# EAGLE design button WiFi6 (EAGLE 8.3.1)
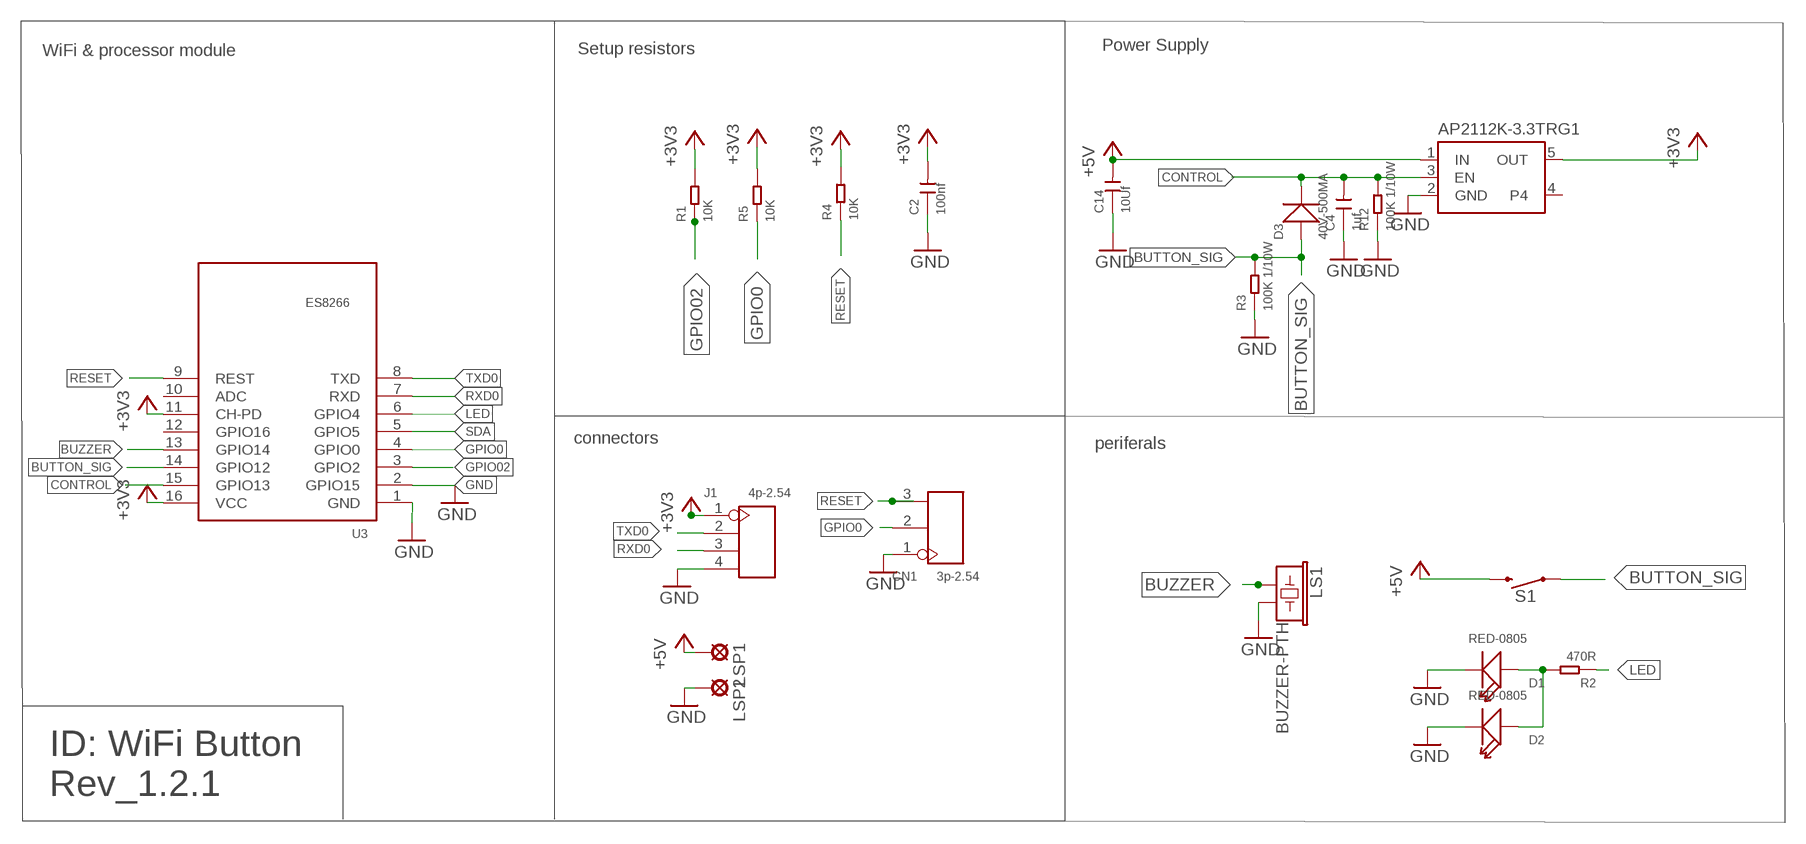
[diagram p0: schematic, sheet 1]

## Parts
AP2112K-3.3TRG1  SPX3819  VREG_SOT23-5  [SOT23-5]
C2  100nf  CERAMIC-100NF-50V-10%-X7R(0603)  [C0603]
C4  1uf  CERAMIC-1UF-25V-10%-X7R(0603)  [C0603]
C14  10Uf  CERAMIC-100NF-50V-10%-X7R(0603)  [C0603]
CN1  3p-2.54  DIP-BLACK-MALE-HEADER-VERT(3P-2.54)  [H3-2.54]
D1  RED-0805  SMD-LED-CLEAR-RED(0805)  [LED-0805]
D2  RED-0805  SMD-LED-CLEAR-RED(0805)  [LED-0805]
D3  40V-500MA  SMD-DIODE-SCHOTTKY-40V-500MA(SOD-123)  [SOD-123]
J1  4p-2.54  DIP-BLACK-FEMALE-HEADER-VERT(4P-2.54)  [H4-2.54]
LS1  BUZZER-PTH  [BUZZER-12MM]
LSP1  SE11  [SE11]
LSP2  SE11  [SE11]
R1  10K  SMD-RES-10K-1%-1/10W(0603)  [R0603]
R2  470R  SMD-RES-470R-5%-1/10W(0603)  [R0603]
R3  100K 1/10W  SMD-RES-100K-5%-1/10W(0603)  [R0603]
R4  10K  SMD-RES-10K-1%-1/10W(0603)  [R0603]
R5  10K  SMD-RES-10K-1%-1/10W(0603)  [R0603]
R12  100K 1/10W  SMD-RES-100K-5%-1/10W(0603)  [R0603]
S1  MOMENTARY-SWITCH-SPST-SMD-6.2MM-TALL  [TACTILE_SWITCH_SMD_6.2MM_TALL]
U3  ES8266  MOUDLE-WIFI-ESP8266-AKX(16P-24X16MM)  [LGA16-2.0-24X16MM]

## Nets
+3V3: AP2112K-3.3TRG1.5(OUT) C2.2 J1.1 R1.2 R4.2 R5.2 U3.11(CH-PD) U3.16(VCC)
+5V: AP2112K-3.3TRG1.1(IN) C14.2 LSP1.MP S1.B2
BUTTON_SIG: D3.+ R3.2 S1.A2 U3.14(GPIO12)
BUZZER: LS1.+ U3.13(GPIO14)
CONTROL: AP2112K-3.3TRG1.3(EN) C4.2 D3.- R12.2 U3.15(GPIO13)
GND: AP2112K-3.3TRG1.2(GND) C2.1 C4.1 C14.1 CN1.1 D1.- D2.- J1.4 LS1.- LSP2.MP R3.1 R12.1 U3.1(GND) U3.2(GPIO15)
GPIO0: CN1.2 R5.1 U3.4(GPIO0)
GPIO02: R1.1 U3.3(GPIO2)
LED: R2.1 U3.6(GPIO4)
N$2: D1.+ D2.+ R2.2
RESET: CN1.3 R4.1 U3.9(REST)
RXD0: J1.3 U3.7(RXD)
SDA: U3.5(GPIO5)
TXD0: J1.2 U3.8(TXD)
Unconnected: AP2112K-3.3TRG1.4 U3.10(ADC) U3.12(GPIO16)

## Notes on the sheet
- Setup resistors | Power Supply
- WiFi & processor module
- connectors
- periferals
- ID: WiFi Button 
  Rev_1.2.1

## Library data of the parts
AP2112K-3.3TRG1 = microbuilder:VREG_SOT23-5: SOT23-5 Fixed Voltage Regulators Part Current Out V Out V In V Dropout θJA (°C/W) TJ (°C) Digikey Part No. ADP121 150mA 3.3V 3.4-5.5V 0.09V @ 150mA -- -- ADP121-AUJZ33R7CT-ND ADP121 150mA 3.0V 3.1-5.5V 0.09V @ 150mA -- -- ADP121-AUJZ30R7CT-ND ADP122 300mA 3.3V 3.4-5.5V 0.085V @ 300mA -- --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
C2 = Seeed-Capacitor:CERAMIC-100NF-50V-10%-X7R(0603): 302010138; MPN: CC0603KRX7R9BB104
C4 = Seeed-Capacitor-2016:CERAMIC-1UF-25V-10%-X7R(0603): 302010139; MPN: CC0603KRX7R8BB105
C14 = Seeed-OPL-Capacitor:CERAMIC-100NF-50V-10%-X7R(0603): 302010138; MPN: CC0603KRX7R9BB104; VALUE: 100nf
CN1 = Seeed-Connector -2016:DIP-BLACK-MALE-HEADER-VERT(3P-2.54): 320020079
D1 D2 = Seeed-LED-2016:SMD-LED-CLEAR-RED(0805): 304090046; MPN: 17-215SURC/S530-A2/TR8
D3 = Seeed-Diode:SMD-DIODE-SCHOTTKY-40V-500MA(SOD-123): 304020012; MPN: B0540W
J1 = Seeed-Connector:DIP-BLACK-FEMALE-HEADER-VERT(4P-2.54): 320030017; MPN: F185-1104A1BSYA1
LS1 = SparkFun-Electromechanical:BUZZER: Buzzer; PROD_ID: COMP-08253; SF_SKU: COM-07950
LSP1 LSP2 = solpad:SE11: SOLDER PAD
R1 R4 R5 = Seeed-Resistor-2016:SMD-RES-10K-1%-1/10W(0603): 301010299; MPN: RC0603FR-0710KL
R2 = Seeed-Resistor-2016:SMD-RES-470R-5%-1/10W(0603): 301010088; MPN: RC0603JR-07470RL
R3 R12 = Seeed-Resistor-2016:SMD-RES-100K-5%-1/10W(0603): 301010089; MPN: RC0603JR-07100KL
S1 = SparkFun-Switches:MOMENTARY-SWITCH-SPST: Momentary Switch (Pushbutton) - SPST; PROD_ID: SWCH-11966; SF_SKU: COM-12992
U3 = Seeed-OPL-Moudle:MOUDLE-WIFI-ESP8266-AKX(16P-24X16MM): 317060011; MPN: ES8266

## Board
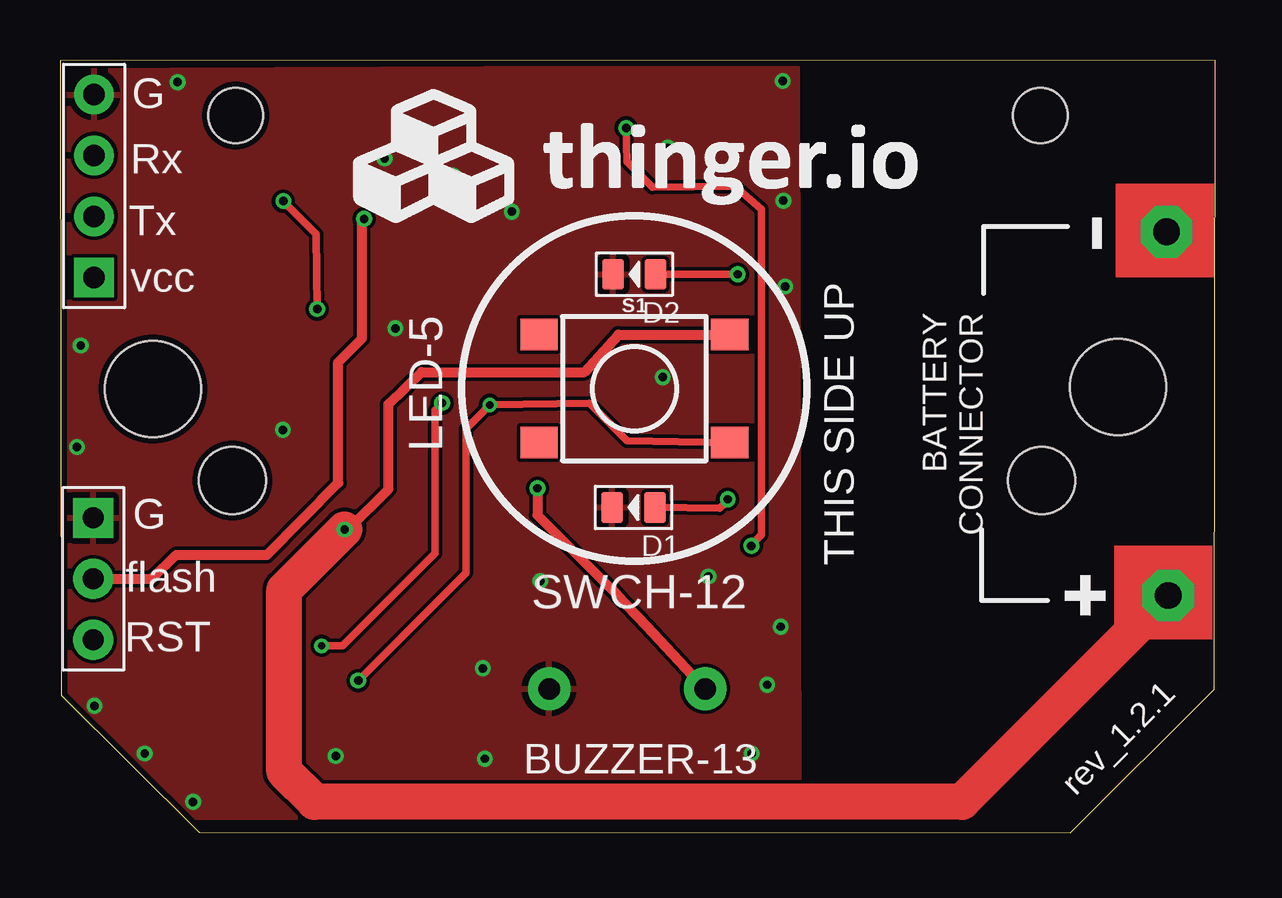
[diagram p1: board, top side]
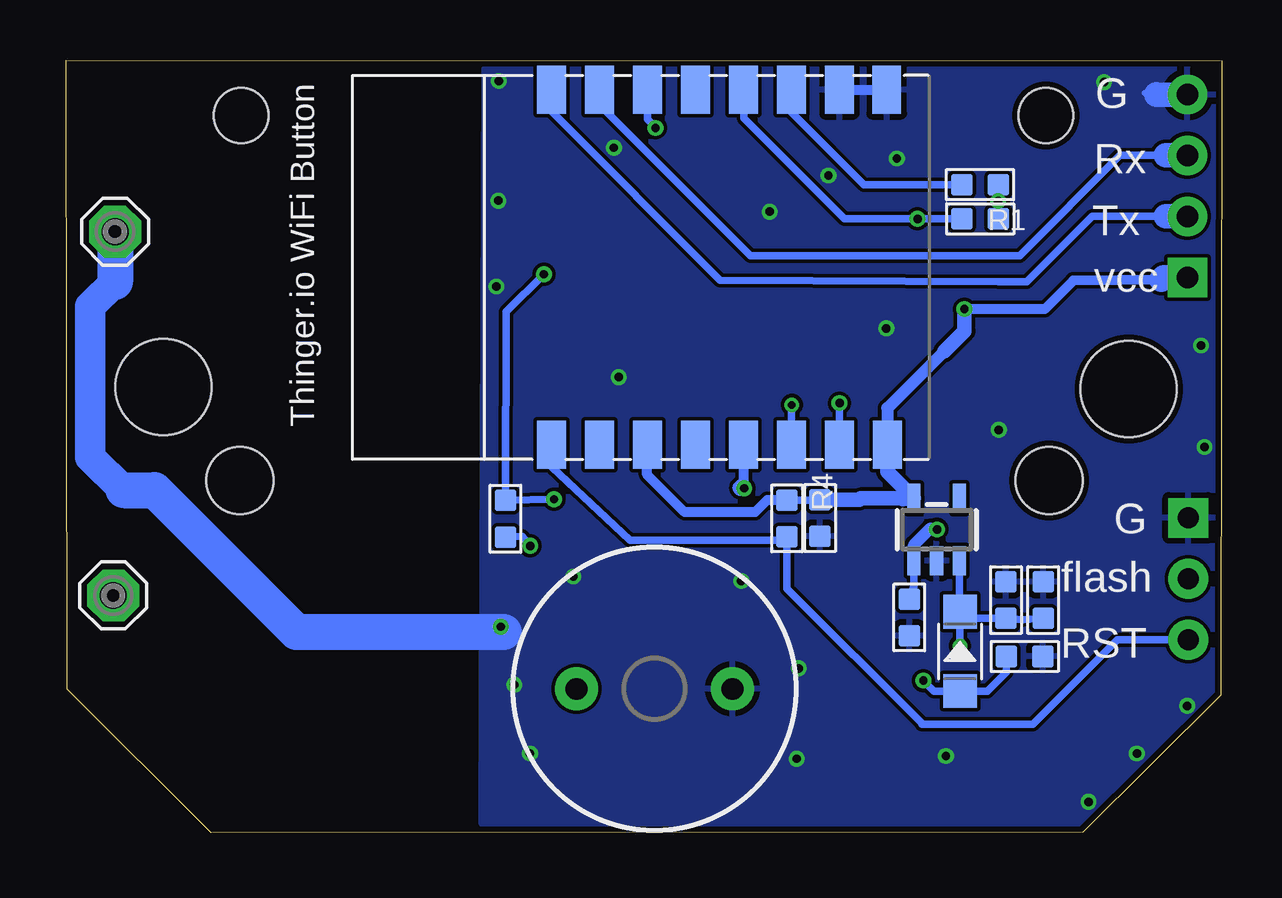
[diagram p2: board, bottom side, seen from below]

Size 48.15 x 32.2 mm. Coordinates in mm from the lower left corner, seen from the top.
Outline: 0,32.18 0.04,5.74 5.79,0.02 42.11,0 48.11,5.99 48.15,32.2 0,32.18
Copper layers (1*16): Top 0.035mm / dielectric 1.5mm / Bottom 0.035mm
Design rules "SeeedStudio_2layer_DRU_no_angle_20140221": minimum track width 6mil, minimum drill 12mil, track to track 6mil, track to pad 6mil, pad to pad 6mil, via to via 6mil, smd to smd 0mil, copper to edge 10mil, drill to drill 10mil, minimum pad ring 10mil, minimum via ring 6mil, stop-mask expansion 2mil, vias tented up to drill 100mil, thermal gap 10mil
Holes 2.8 mm at 7.19,14.69 40.92,14.69
Holes 2.29 mm at 7.33,29.89 40.86,29.89
Holes 4 mm at 3.87,18.5 44.11,18.57

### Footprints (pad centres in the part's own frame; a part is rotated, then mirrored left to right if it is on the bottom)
SOT23-5 = smd 0.55 x 1.2: 1 -0.95,-1.3; 2 0,-1.3; 3 0.95,-1.3; 4 0.95,1.3; 5 -0.95,1.3
C0603 = smd 0.889 x 0.889: 1 0,0.762; 2 0,-0.762
H3-2.54 = drill 0.889 pad 1.651 square: 1 0,2.54 | drill 0.889 pad 1.651: 2 0,0; 3 0,-2.54
LED-0805 = smd 0.889 x 1.27: + -0.889,0; - 0.889,0
SOD-123 = smd 1.397 x 1.397: + -1.651,0; - 1.651,0
H4-2.54 = drill 0.889 pad 1.651 square: 1 0,3.81 | drill 0.889 pad 1.651: 2 0,1.27; 3 0,-1.27; 4 0,-3.81
BUZZER-12MM = drill 0.9 pad 1.778: + 3.25,0; - -3.25,0
SE11 = drill 1.118 pad 2.159 octagon: MP 0,0
R0603 = smd 0.889 x 0.889: 1 0,0.762; 2 0,-0.762
TACTILE_SWITCH_SMD_6.2MM_TALL = smd 1.55 x 1.3: A1 -3.975,-2.25; A2 3.975,-2.25; B1 -3.975,2.25; B2 3.975,2.25
LGA16-2.0-24X16MM = smd 2 x 1.2: 1 7.4,-10.27; 2 7.4,-8.3; 3 7.4,-6.3; 4 7.4,-4.3; 5 7.4,-2.3; 6 7.4,-0.3; 7 7.4,1.7; 8 7.4,3.7; 9 -7.4,3.7; 10 -7.4,1.7; 11 -7.4,-0.3; 12 -7.4,-2.3; 13 -7.4,-4.3; 14 -7.4,-6.3; 15 -7.4,-8.3; 16 -7.4,-10.3

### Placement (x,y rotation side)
AP2112K-3.3TRG1  11.88,12.64 0 bottom
C2  16.74,13.12 180 bottom
C4  8.99,9.7 0 bottom
C14  13.01,8.98 180 bottom
CN1  1.39,10.59 0 top
D1  23.9,13.56 180 top
D2  23.94,23.28 180 top
D3  10.9,7.56 90 bottom
J1  1.42,26.96 180 top
LS1  23.64,6 180 bottom
LSP1  46.2,9.89 0 bottom
LSP2  46.12,25.05 0 bottom
R1  10.07,27.01 90 bottom
R2  29.86,13.09 180 bottom
R3  8.21,7.35 270 bottom
R4  18.11,13.1 180 bottom
R5  10.06,25.58 90 bottom
R12  7.44,9.7 0 bottom
S1  23.94,18.51 0 top
U3  24.23,23.57 90 bottom

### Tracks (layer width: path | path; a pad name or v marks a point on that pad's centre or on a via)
+3V3  (via drill 0.35)
  Top 0.305: v10.72,21.83 10.68,24.95 v9.31,26.32
  Bottom 0.203: U3.16 13.93,15.61
  Bottom 0.254: 2.95,22.95 J1.1
  Bottom 0.305: C2.2 16.76,13.86 16.76,13.87 R4.2 | U3.16 13.93,15.56 | R5.2 v9.31,26.32 R1.2
  Bottom 0.406: 2.51,23.05 6.19,23.01 7.37,21.83 v10.72,21.83 | R4.2 18.95,13.87 19.45,13.37 22.38,13.37 23.94,14.93 23.94,16.16 U3.11
  Bottom 0.508: U3.16 13.93,17.7 11.56,20.07 | v10.72,21.83 10.73,21.49
  Bottom 0.61: 14.23,15.86 U3.16 13.93,15.04 AP2112K-3.3TRG1.5 | AP2112K-3.3TRG1.5 13.28,13.89 | C2.2 15.1,13.88 15.05,13.94 AP2112K-3.3TRG1.5 | 11.56,20.07 10.72,20.91 v10.72,21.83
  Bottom 1.016: J1.1 2.41,23.15 2.51,23.05
+5V  (via drill 0.35)
  Top 0.406: v11.86,12.65 12.02,12.65 13.69,14.32 13.69,17.87 15.06,19.2 21.86,19.2 23.27,20.76 S1.B2
  Top 1.016: 45.5,9.19 LSP1.MP
  Top 1.5: LSP1.MP 37.6,1.29 10.61,1.29 9.35,2.55 9.35,10.13 v11.86,12.65
  Bottom 0.305: AP2112K-3.3TRG1.1 12.83,10.27 C14.2
  Bottom 0.508: AP2112K-3.3TRG1.1 12.82,11.35 12.82,12 12.13,12.68 v11.86,12.65
BUTTON_SIG  (via drill 0.3, 0.35)
  Top 0.305: 27.74,16.57 S1.A2 23.64,16.34 22.07,17.91 v17.92,17.84 16.93,16.85 16.93,10.85 v12.43,6.35
  Bottom 0.305: v12.43,6.35 12,5.91 D3.+ | D3.+ 11.02,5.87 | D3.+ | R3.2 8.97,6.7 9.77,5.9 10.89,5.9 D3.+ | U3.14 17.93,17.82 v17.92,17.84
BUZZER  (via drill 0.35)
  Top 0.406: 23.2,9.94 22.95,10.21 | 23.2,9.94 24.48,8.61 LS1.+ | v19.9,14.36 19.9,13.24 23.2,9.94
  Bottom 0.406: U3.13 19.93,14.29 19.94,14.28 arc323 v19.9,14.36
CONTROL  (via drill 0.3, 0.35)
  Top 0.305: v15.93,17.91 15.64,17.62 15.64,11.66 11.78,7.8 v10.91,7.79
  Bottom 0.305: U3.15 15.93,17.76 15.85,17.84 v15.93,17.91 | 7.49,8.89 R12.2 8.28,8.89 C4.2 10.62,8.94 D3.- | D3.- 10.9,8.68 v10.91,7.79 | AP2112K-3.3TRG1.3 10.93,9.24 D3.-
GND  (via drill 0.35)
  Bottom 0.254: 2.73,30.78 3.22,30.82
  Bottom 0.406: U3.2 U3.1
  Bottom 1.016: J1.4 2.72,30.77 2.73,30.78
  Bottom 1.27: 46.12,22.96 47.15,21.94 47.15,15.66 45.77,14.28
  Bottom 1.5: LSP2.MP 46.12,22.96 | 45.77,14.28 44.48,14.28 38.57,8.38 29.92,8.38
  other vias: 30.15,26.34 30.13,31.33 13.53,28.09 18.84,25.88 13.98,21.02 30.23,22.76 17.63,6.86 17.71,3.09 28.83,3.31 16.39,27.39 25.33,28.55 11.49,3.2 3.53,3.31 27.03,10.68 20.02,10.49 25.12,18.99 30.04,8.59 9.29,16.79 5.55,1.29 1.44,5.29 0.71,16.08 0.86,20.31 4.9,31.28 29.48,6.17
  pour Bottom: 0.19,32 0.32,0.36 30.84,0.36 30.73,31.84
  pour Top: 0.23,31.73 0.12,5.85 5.62,0.66 30.81,0.71 30.73,31.87
GPIO0  (via drill 0.35)
  Top 0.305: 12.51,25.47 12.69,25.64
  Top 0.406: v12.68,25.59 12.69,25.6 12.69,25.64 12.59,25.54 12.59,20.61 11.6,19.62 11.6,14.59 8.63,11.58 4.85,11.58 3.83,10.59 CN1.2
  Bottom 0.305: R5.1 12.54,25.59 v12.68,25.59 15.68,25.59 15.69,25.59 | 19.89,30.92 U3.4 19.91,30.94 19.91,29.77 15.73,25.59 15.69,25.59 | 15.69,25.59 15.54,25.59
GPIO02
  Bottom 0.305: R1.1 14.91,27.01 18,30.1 18,30.9 U3.3
LED  (via drill 0.35)
  Top 0.305: v23.6,29.37 23.64,27.96 24.7,26.9 28.13,26.93 29.24,25.98 29.24,12.42 28.82,12 v28.82,11.96
  Bottom 0.305: U3.6 23.93,29.74 v23.6,29.37 23.45,29.26 | v28.82,11.96 29.16,12.36 R2.1
N$2  (via drill 0.35)
  Top 0.305: D1.+ 27.49,13.52 27.87,13.87 v27.83,13.9 | D2.+ v28.25,23.28
  Bottom 0.305: v28.25,23.28 29.82,21.71 R2.2 v27.83,13.9
RESET
  Bottom 0.305: U3.9 27.9,16.14 27.9,15.24 24.67,12.19 18.27,12.19 R4.1 18.11,10.17 12.5,4.56 12.5,4.53 7.86,4.53 4.35,8.05 CN1.3
RXD0
  Bottom 0.254: J1.3
  Bottom 0.305: U3.7 25.96,30.94 25.87,30.85 25.8,30.21 19.63,24.05 8.42,24.05 4.24,28.23 J1.3
  Bottom 1.016: J1.3 2.34,28.23
TXD0
  Bottom 0.305: 27.91,30.62 27.91,30.04 20.91,23.04 9.31,22.96 8.11,22.96 5.39,25.69 2.08,25.69 | 27.91,30.62 27.91,30.95 U3.8 | 27.93,30.6 27.91,30.62
  Bottom 1.016: J1.2 2.08,25.69 2.33,25.69
(copper drawn outside any net)
  shapes: Top area x2

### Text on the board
tNames: G | Rx | Tx | - | vcc | LED-5 | BATTERY / CONNECTOR | G | THIS SIDE UP | flash | SWCH-12 | RST | rev_1.2.1 | BUZZER-13
bNames: G | Rx | Tx | vcc | Thinger.io WiFi Button | G | flash | RST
